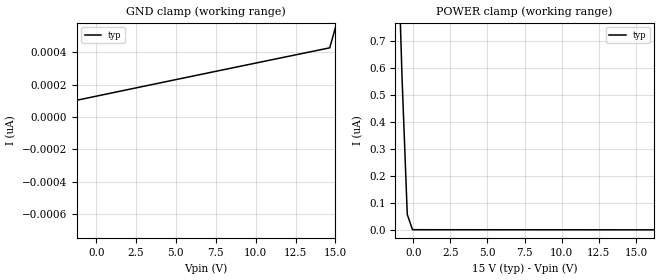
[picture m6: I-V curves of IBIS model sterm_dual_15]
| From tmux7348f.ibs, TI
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| sterm_dual_15
[Model]   sterm_dual_15
Model_type   Terminator
|   typ   min   max
C_comp   1.598234e-12   NA   NA
[Voltage Range]   15   NA   NA
[Temperature Range]   27   NA   NA
[Power Clamp Reference]   15   NA   NA
[GND Clamp Reference]   0   NA   NA
[GND Clamp]
|   Voltage   I(typ)   I(min)   I(max)
-20V      -19.25uA   NA         NA
-15.05V   -1.625nA   NA         NA
-14.7V    -176.6pA   NA         NA
14.65V    428.4pA    NA         NA
15V       552.4pA    NA         NA
[POWER Clamp]
|   Voltage   I(typ)   I(min)   I(max)
-5V       8.864uA    NA         NA
-1.111V   1.206uA    NA         NA
-757.6mV  567.2nA    NA         NA
-404mV    57.08nA    NA         NA
-50.5mV   565.4pA    NA         NA
30V       -515.6pA   NA         NA
